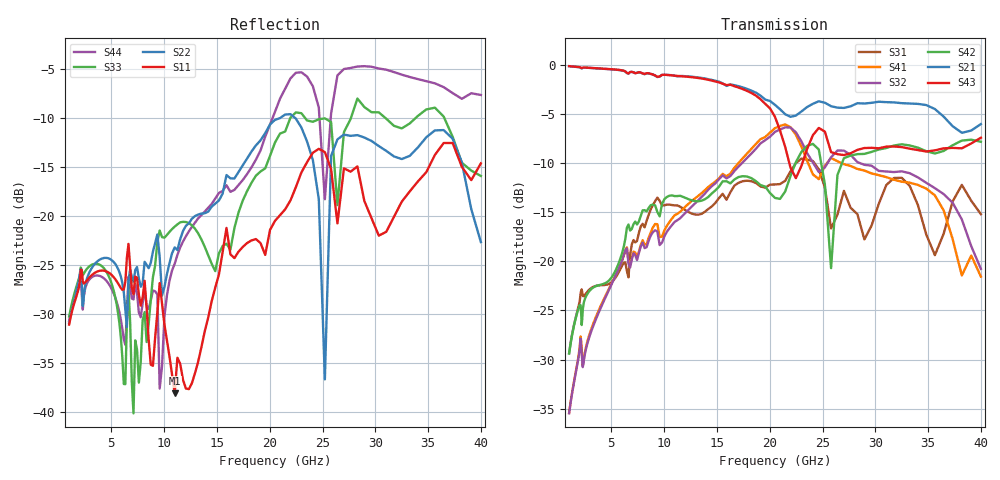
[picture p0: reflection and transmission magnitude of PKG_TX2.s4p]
! Created Mon Sep 18 16:08:56 2017
# hz S ma R 50
! 4 Port Network Data from SP1.SP block
! freq  magS11  angS11  magS12  angS12  magS13  angS13  magS14  angS14
!  magS21  angS21  magS22  angS22  magS23  angS23  magS24  angS24
!  magS31  angS31  magS32  angS32  magS33  angS33  magS34  angS34
!  magS41  angS41  magS42  angS42  magS43  angS43  magS44  angS44
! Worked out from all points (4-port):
!   161 points, 1 GHz to 40 GHz, reference 50 ohm
!   strongest paths, dB at 1 GHz, 2.515 GHz, 6.325 GHz, 15.91 GHz, 40 GHz:
!     S43: -0.2, -0.3, -0.7, -2.1, -7.4
!     S21: -0.2, -0.3, -0.7, -2.2, -6.0
!     S42: -29.4, -23.8, -17.7, -11.9, -7.8
!     S32: -35.5, -29.3, -18.9, -11.6, -20.8
!     S41: -35.4, -29.1, -18.9, -11.3, -21.5
!     S31: -29.3, -23.4, -20.1, -13.7, -15.2
!   lowest |S11| = -38.1 dB at 11 GHz (marker M1), VSWR 1.03, Z = 50.9 - j0.924 ohm
!   |S11| at or under -10 dB: start of sweep to end of sweep
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1e9  0.02797 44.9  0.9822 -25.6  0.0341 54.1  0.01696 -120.4
     0.9822 -25.6  0.02858 34.1  0.01687 -120.3  0.03398 71.2
     0.0341 54.1  0.01687 -120.3  0.03071 42.3  0.9827 -25.0
     0.01696 -120.4  0.03398 71.2  0.9827 -25.0  0.02918 42.3
6.324555e9  0.04634 -16.6  0.9227 -159.3  0.09873 157.6  0.1137 105.9
            0.9227 -159.3  0.03319 -87.6  0.1135 109.4  0.1301 61.8
            0.09873 157.6  0.1135 109.4  0.01388 -27.6  0.924 -156.0
            0.1137 105.9  0.1301 61.8  0.924 -156.0  0.02205 -10.0
1.099864e10  0.01247 -46.8  0.8789 86.5  0.1926 -18.9  0.1716 -10.4
             0.8789 86.5  0.06931 -74.6  0.1588 -0.7  0.2146 14.5
             0.1926 -18.9  0.1588 -0.7  0.08854 -63.0  0.8795 91.7
             0.1716 -10.4  0.2146 14.5  0.8795 91.7  0.05718 1.0
1.784881e10  0.07295 -51.4  0.7529 -86.4  0.2571 38.6  0.3531 168.7
             0.7529 -86.4  0.1972 -117.8  0.3353 -174.3  0.2699 -44.4
             0.2571 38.6  0.3353 -174.3  0.1341 -22.2  0.7357 -84.1
             0.3531 168.7  0.2699 -44.4  0.7357 -84.1  0.164 -110.1
2.522333e10  0.2126 -50.6  0.6405 105.1  0.2376 22.8  0.306 -49.4
             0.6405 105.1  0.01469 160.0  0.3001 -26.5  0.2463 -24.2
             0.2376 22.8  0.3001 -26.5  0.3165 -5.2  0.4566 116.6
             0.306 -49.4  0.2463 -24.2  0.4566 116.6  0.1222 8.9
3.326266e10  0.134 -20.9  0.6345 -91.7  0.2416 10.1  0.2512 84.9
             0.6345 -91.7  0.2035 -48.9  0.2807 113.1  0.3884 -28.4
             0.2416 10.1  0.2807 113.1  0.298 15.4  0.374 -46.3
             0.2512 84.9  0.3884 -28.4  0.374 -46.3  0.5146 -37.1
4e10  0.1864 79.7  0.4988 110.6  0.1737 29.3  0.08368 -69.2
      0.4988 110.6  0.07381 -104.0  0.09153 -58.3  0.4054 -66.7
      0.1737 29.3  0.09153 -58.3  0.1606 -165.2  0.4252 169.7
      0.08368 -69.2  0.4054 -66.7  0.4252 169.7  0.4165 -69.6
